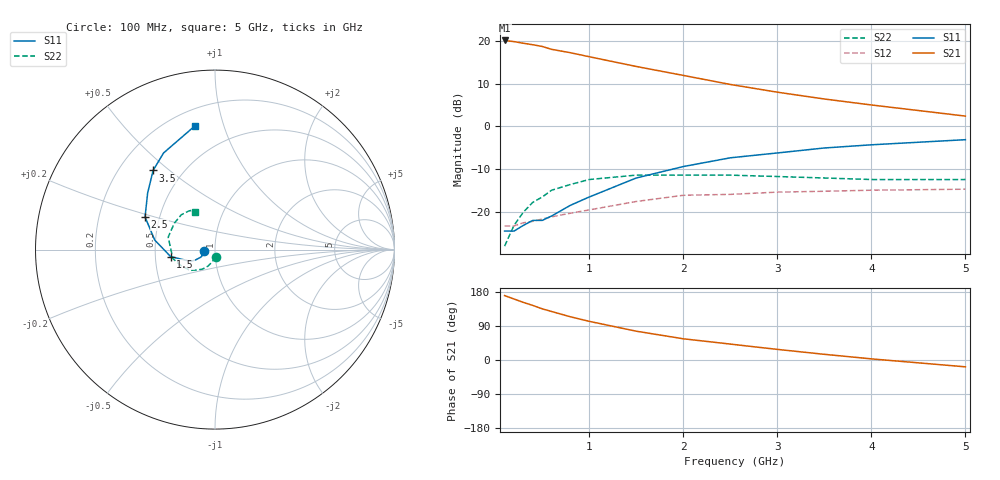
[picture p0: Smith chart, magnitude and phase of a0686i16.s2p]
!  MSA-0686 S AND NOISE PARAMETERS
!  Id=16mA  LAST UPDATED 07-22-92
# ghz s ma r 50
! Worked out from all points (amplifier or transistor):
!   15 points, 100 MHz to 5 GHz, reference 50 ohm
!   highest |S21| = 20.1 dB at 100 MHz (marker M1)
!   |S21| within 3 dB of that: start of sweep to 829.4 MHz
!   unconditionally stable (mu >= 1): start of sweep to end of sweep
!   at 300 MHz: K = 1.05, MAG = 19.6 dB, |S12| = -22.5 dB
!   at 1 GHz: K = 1.01, MAG = 17.2 dB, |S12| = -19.5 dB
!   at 5 GHz: K = 1.20, MAG = 5.8 dB, |S12| = -14.7 dB
!   lowest NFmin = 2.90 dB at 100 MHz
!   S11 on the Smith chart (normalised r, x): 100 MHz: 0.89, -0.01; 1.5 GHz: 0.60, -0.05; 2.5 GHz: 0.41, +0.19; 3.5 GHz: 0.34, +0.44; 5 GHz: 0.30, +0.81
0.1  0.06 -175.0  10.08 170.0  0.069 4.0  0.04 -84.0
0.2  0.06 -169.0  9.77 161.0  0.069 8.0  0.07 -103.0
0.3  0.07 -164.0  9.35 152.0  0.075 13.0  0.1 -113.0
0.4  0.08 -158.0  8.98 144.0  0.078 16.0  0.13 -123.0
0.5  0.08 -154.0  8.58 135.0  0.083 18.0  0.15 -131.0
0.6  0.09 -152.0  7.94 128.0  0.088 21.0  0.18 -140.0
0.8  0.12 -152.0  7.25 114.0  0.097 25.0  0.21 -155.0
1  0.15 -154.0  6.51 102.0  0.106 25.0  0.24 -168.0
1.5  0.25 -171.0  5.01 76.0  0.133 22.0  0.27 165.0
2  0.34 171.0  3.94 56.0  0.157 19.0  0.27 147.0
2.5  0.43 155.0  3.09 42.0  0.161 16.0  0.27 134.0
3  0.49 140.0  2.51 28.0  0.171 11.0  0.26 124.0
3.5  0.56 128.0  2.09 15.0  0.175 6.0  0.25 118.0
4  0.61 118.0  1.78 3.0  0.18 3.0  0.24 115.0
5  0.7 99.0  1.32 -18.0  0.185 -2.0  0.24 118.0
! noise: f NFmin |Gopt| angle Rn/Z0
0.1  2.9  0.12  4  0.4
0.5  3  0.1  16  0.4
1  3.1  0.06  40  0.38
2  3.5  0.07  -161  0.34
